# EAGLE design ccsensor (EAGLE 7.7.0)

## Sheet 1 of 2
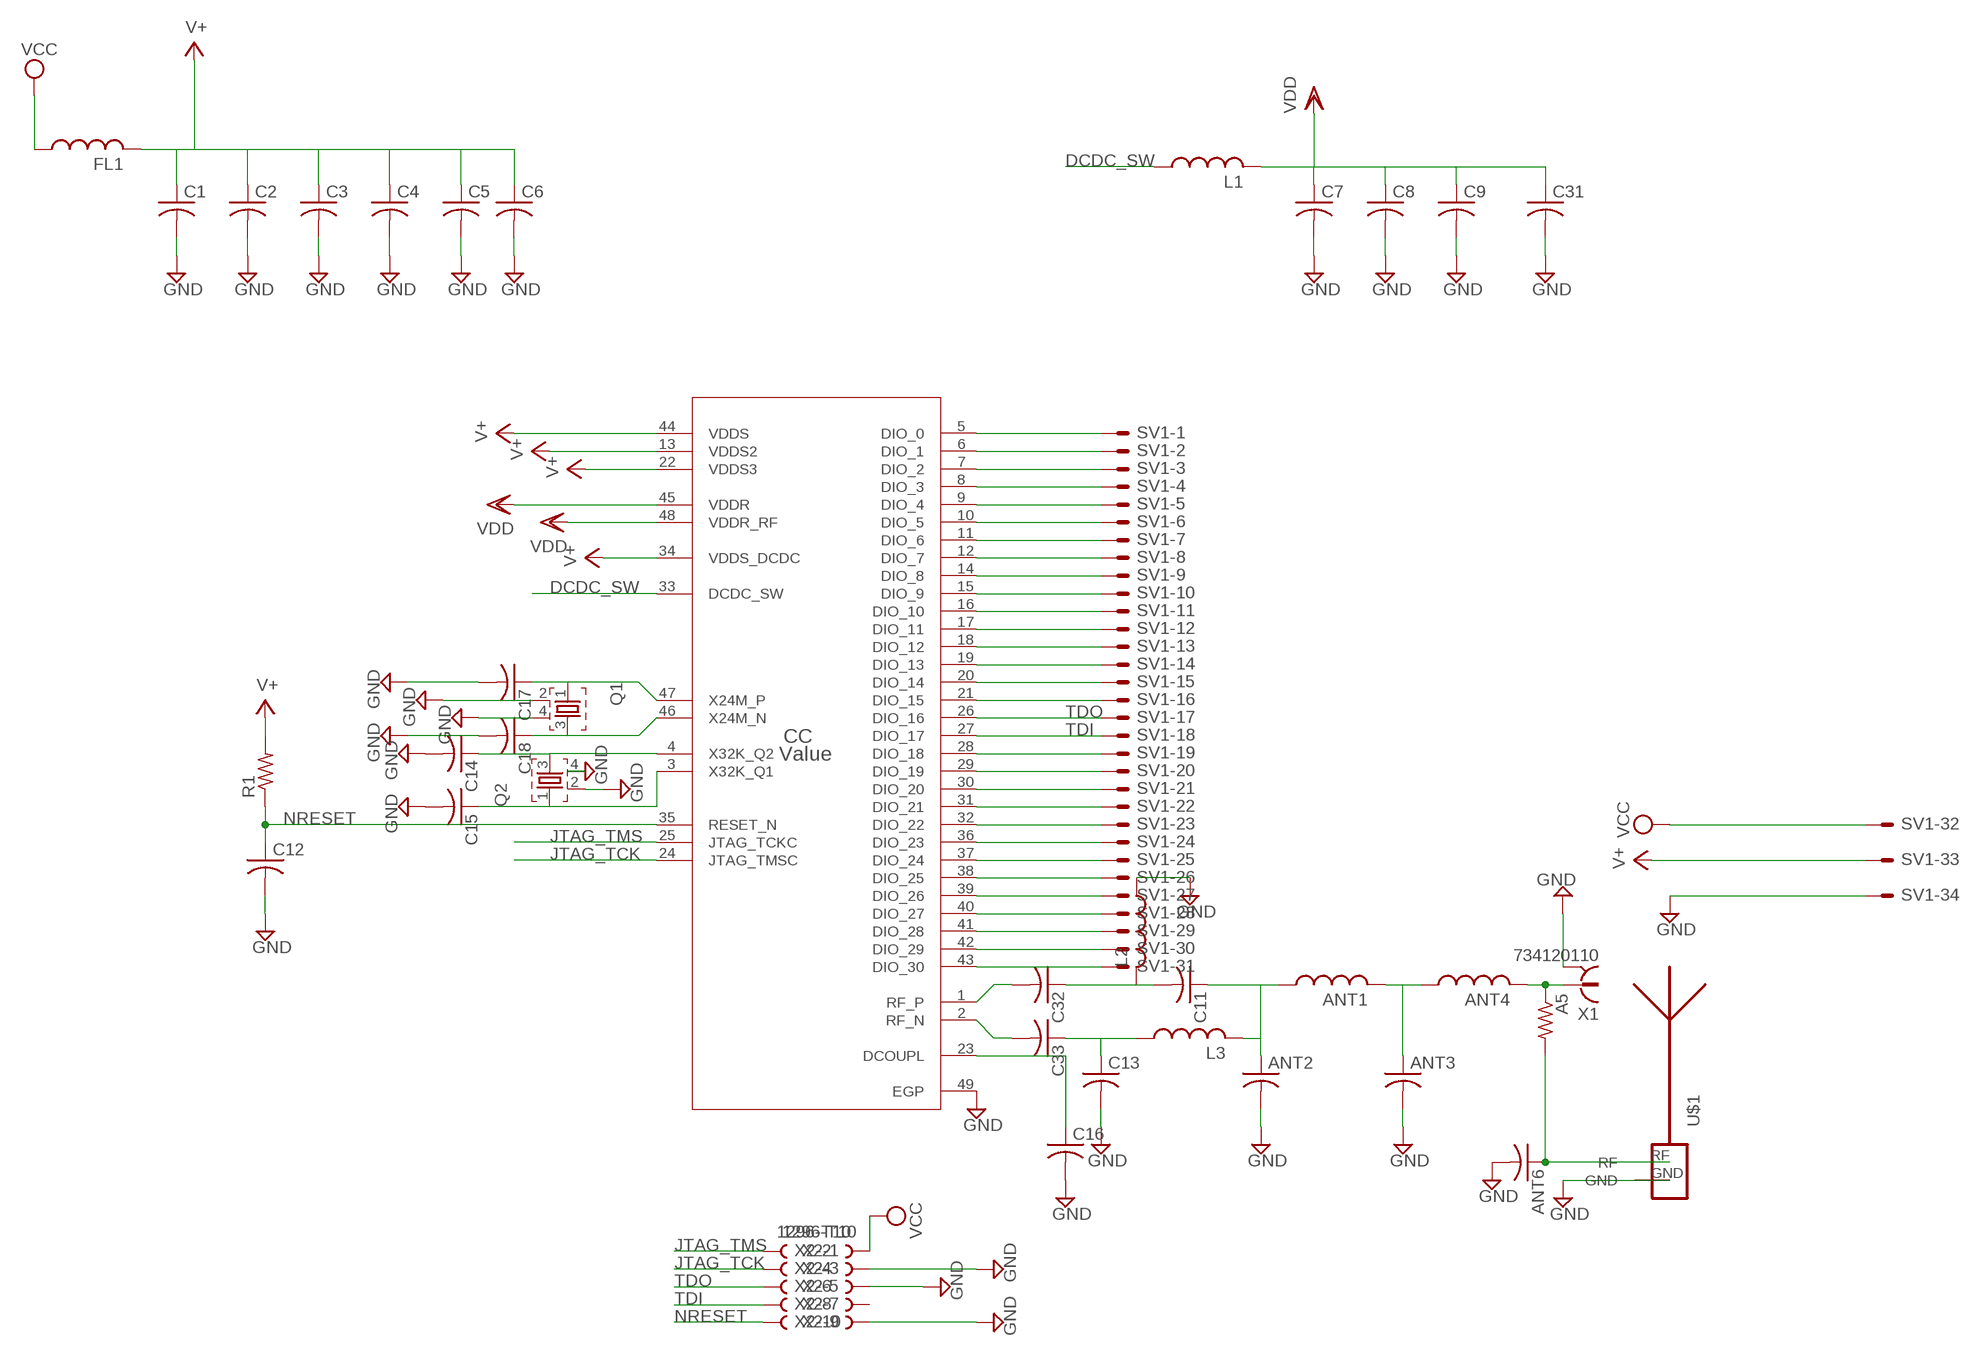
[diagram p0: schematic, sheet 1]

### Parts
A5  R-US_R0402  [R0402]
ANT1  L-USL2012C  [L2012C]
ANT2  C-USC0402  [C0402]
ANT3  C-USC0402  [C0402]
ANT4  L-USL2012C  [L2012C]
ANT6  C-USC0402  [C0402]
C1  C-USC0402  [C0402]
C2  C-USC0402  [C0402]
C3  C-USC0402  [C0402]
C4  C-USC0402  [C0402]
C5  C-USC0603  [C0603]
C6  C-USC0402  [C0402]
C7  C-USC0402  [C0402]
C8  C-USC0402  [C0402]
C9  C-USC0402  [C0402]
C11  C-USC0402  [C0402]
C12  C-USC0402  [C0402]
C13  C-USC0402  [C0402]
C14  C-USC0402  [C0402]
C15  C-USC0402  [C0402]
C16  C-USC0402  [C0402]
C17  C-USC0402  [C0402]
C18  C-USC0402  [C0402]
C31  C-USC0402  [C0402]
C32  C-USC0402  [C0402]
C33  C-USC0402  [C0402]
CC  Value  CC2650F128RGZR  [RGZ0048A]
FL1  L-USL2012C  [L2012C]
L1  L-USL2012C  [L2012C]
L2  L-USL2012C  [L2012C]
L3  L-USL2012C  [L2012C]
Q1  FA-20H  [FA-20H]
Q2  FA-20H  [FA-20H]
R1  R-US_R0402  [R0402]
SV1  ML34E  [ML34]
U$1  ANTENNA_1LEFT  [SWRA117D_LEFT]
X1  734120110  [734120110]
X2  1296-T10  [1296-10]

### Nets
DCDC_SW: CC.33(DCDC_SW) L1.1
GND: ANT2.2 ANT3.2 ANT6.2 C1.2 C2.2 C3.2 C4.2 C5.2 C6.2 C7.2 C8.2 C9.2 C12.2 C13.2 C14.2 C15.2 C16.2 C17.2 C18.2 C31.2 CC.49(EGP) L2.1 Q1.2 Q1.4 Q2.2 Q2.4 SV1.34 U$1.GND X1.S@1 X1.S@2 X1.S@3 X2.3 X2.5 X2.9
JTAG_TCK: CC.24(JTAG_TMSC) X2.4
JTAG_TMS: CC.25(JTAG_TCKC) X2.2
N$1: C18.1 CC.46(X24M_N) Q1.3
N$2: C17.1 CC.47(X24M_P) Q1.1
N$3: C32.2 CC.1(RF_P)
N$4: C15.1 CC.3(X32K_Q1) Q2.1
N$5: C14.1 CC.4(X32K_Q2) Q2.3
N$6: C33.2 CC.2(RF_N)
N$7: C11.2 C32.1 L2.2
N$8: C13.1 C33.1 L3.1
N$9: ANT1.1 ANT2.1 C11.1 L3.2
N$10: ANT1.2 ANT3.1 ANT4.1
N$11: A5.1 ANT4.2 X1.1
N$12: CC.5(DIO_0) SV1.1
N$13: CC.6(DIO_1) SV1.2
N$14: CC.7(DIO_2) SV1.3
N$15: CC.8(DIO_3) SV1.4
N$16: CC.9(DIO_4) SV1.5
N$17: CC.10(DIO_5) SV1.6
N$18: CC.11(DIO_6) SV1.7
N$19: CC.12(DIO_7) SV1.8
N$20: CC.14(DIO_8) SV1.9
N$21: CC.15(DIO_9) SV1.10
N$22: CC.16(DIO_10) SV1.11
N$23: CC.17(DIO_11) SV1.12
N$24: CC.18(DIO_12) SV1.13
N$25: CC.19(DIO_13) SV1.14
N$26: CC.20(DIO_14) SV1.15
N$27: CC.21(DIO_15) SV1.16
N$28: A5.2 ANT6.1 U$1.RF
N$29: C16.1 CC.23(DCOUPL)
N$30: CC.28(DIO_18) SV1.19
N$31: CC.29(DIO_19) SV1.20
N$32: CC.30(DIO_20) SV1.21
N$33: CC.31(DIO_21) SV1.22
N$34: CC.32(DIO_22) SV1.23
N$35: CC.36(DIO_23) SV1.24
N$36: CC.37(DIO_24) SV1.25
N$37: CC.38(DIO_25) SV1.26
N$38: CC.39(DIO_26) SV1.27
N$39: CC.40(DIO_27) SV1.28
N$40: CC.41(DIO_28) SV1.29
N$41: CC.42(DIO_29) SV1.30
N$42: CC.43(DIO_30) SV1.31
NRESET: C12.1 CC.35(RESET_N) R1.1 X2.10
TDI: CC.27(DIO_17) SV1.18 X2.8
TDO: CC.26(DIO_16) SV1.17 X2.6
V+: C1.1 C2.1 C3.1 C4.1 C5.1 C6.1 CC.13(VDDS2) CC.22(VDDS3) CC.34(VDDS_DCDC) CC.44(VDDS) FL1.2 R1.2 SV1.33
VCC: FL1.1 SV1.32 X2.1
VDD: C7.1 C8.1 C9.1 C31.1 CC.45(VDDR) CC.48(VDDR_RF) L1.2
Unconnected: X2.7

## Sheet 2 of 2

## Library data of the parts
A5 R1 = rcl:R-US_: RESISTOR, American symbol; OC_NEWARK: unknown
ANT1 ANT4 FL1 L1-L3 = rcl:L-US: INDUCTOR, American symbol; OC_NEWARK: unknown
ANT2 ANT3 ANT6 C1-C9 C11-C18 C31-C33 = rcl:C-US: CAPACITOR, American symbol; OC_NEWARK: unknown
CC = CC2650F128RGZR:CC2650F128RGZR; ALTERNATEPARTNUMBER: CC2650F128RGZT; APPLICATION_BUILDNUMBER: *; COMPTYPE: IC; MANUFACTURER: Texas Instruments; MOUNTTYPE: SMT; OC_NEWARK: unknown; PACKAGEREFERENCE: RGZ0048A; PARTNUMBER: CC2650F128RGZR; PIN_COUNT: 49; REFDES: RefDes; ROHS: Y; TYPE: TYPE
Q1 Q2 = crystal:FA-: MHz RANGE CRYSTAL UNIT Source: Epson Toyocom; OC_NEWARK: unknown
SV1 = con-ml:ML34E: HARTING; OC_FARNELL: unknown; OC_NEWARK: unknown
U$1 = ant-planar-1:ANTENNA_1; OC_NEWARK: unknown
X1 = con-coax:734120110: MICRO COAXIAL CONNECTOR RECEPTACLE VERTICAL; OC_NEWARK: unknown
X2 = con-leotronics:1296-T10: 1.27mm SINGLE ROW FEMALE SOCKET Source: http://www.leotronics.co.uk/Conexcon/Data%20Sheets/sec.%20A/1296ing.pdf; OC_FARNELL: unknown; OC_NEWARK: unknown

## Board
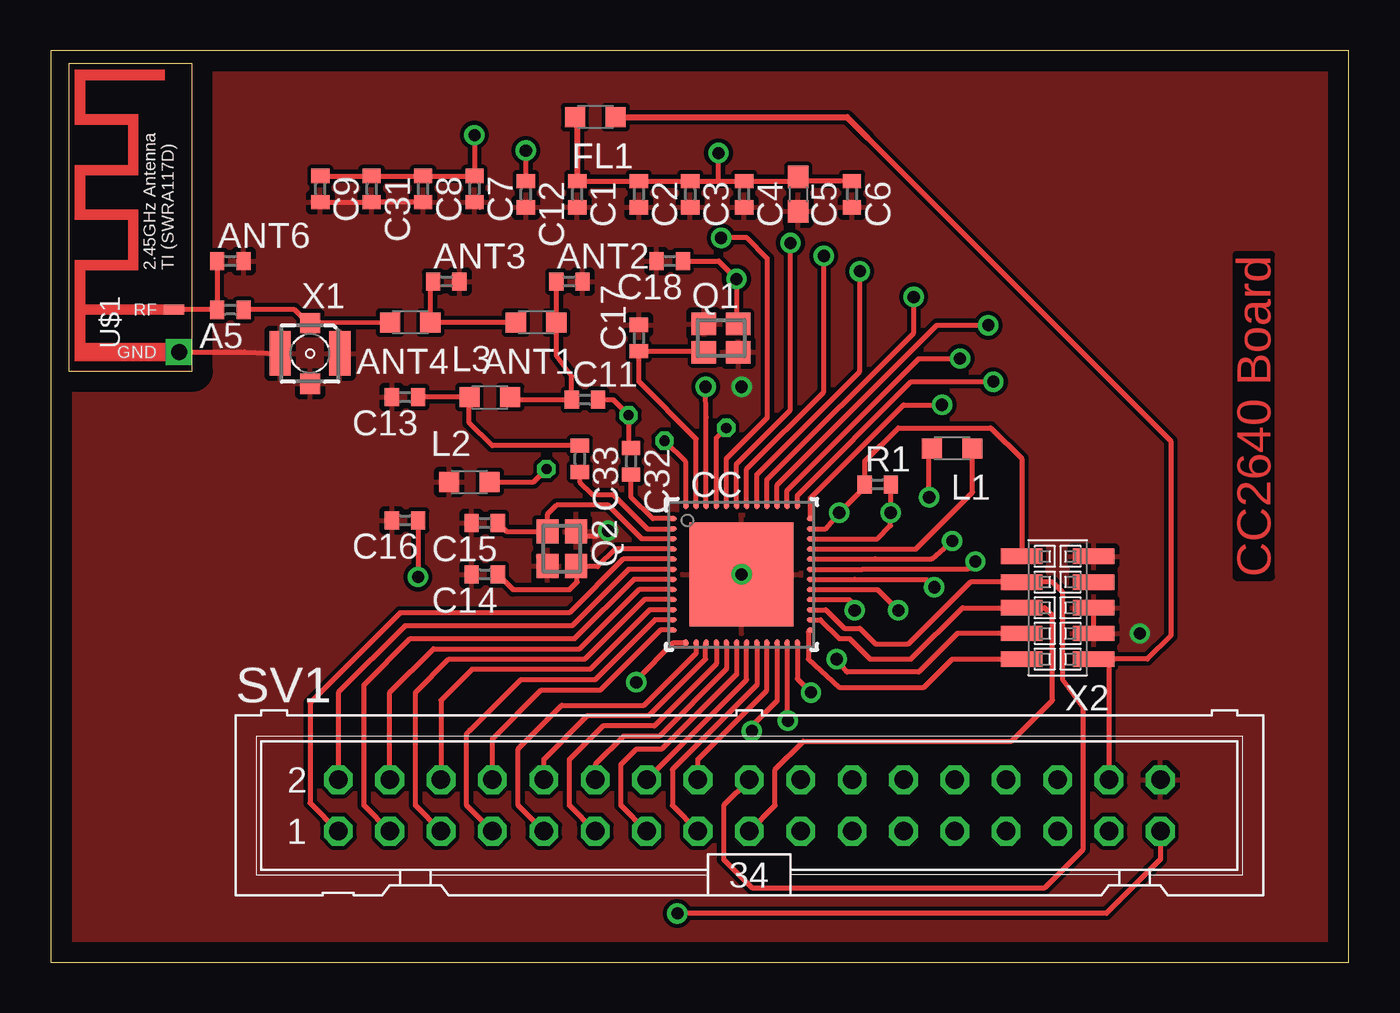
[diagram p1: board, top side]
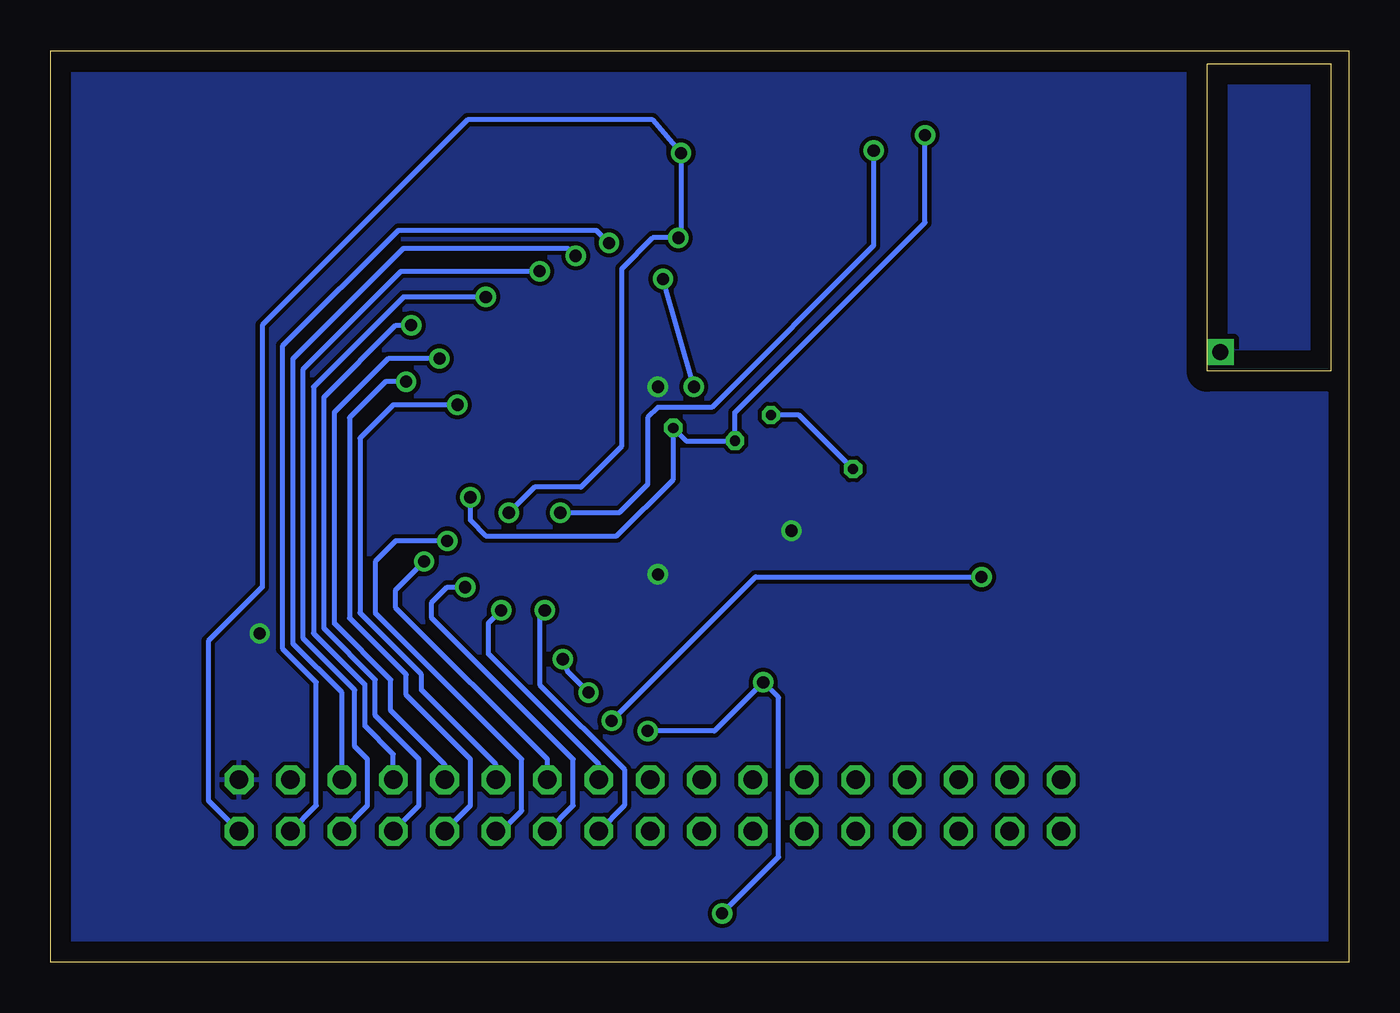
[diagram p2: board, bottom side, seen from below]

Size 64.19 x 45.07 mm. Coordinates in mm from the lower left corner, seen from the top.
Outline: 0,0 64.19,0 64.19,45.07 0,45.07 0,0
Copper layers (1*16): Top 0.035mm / dielectric 1.5mm / Bottom 0.035mm
Design rules "default *": minimum track width 10mil, minimum drill 24mil, track to track 8mil, track to pad 8mil, pad to pad 8mil, via to via 8mil, smd to smd 8mil, copper to edge 40mil, drill to drill 8mil, minimum pad ring 10mil, minimum via ring 8mil, stop-mask expansion 4mil, vias tented up to drill 0mil, thermal gap 10mil

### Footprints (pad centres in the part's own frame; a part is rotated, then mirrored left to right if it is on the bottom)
R0402 = smd 0.7 x 0.9: 1 -0.65,0; 2 0.65,0
L2012C = smd 1 x 1: 1 -1,0; 2 1,0
C0402 = smd 0.7 x 0.9: 1 -0.65,0; 2 0.65,0
C0603 = smd 1.1 x 1: 1 -0.85,0; 2 0.85,0
RGZ0048A = smd 0.36 x 0.24: 1 -3.4,2.75; 2 -3.4,2.25; 3 -3.4,1.75; 4 -3.4,1.25; 5 -3.4,0.75; 6 -3.4,0.25; 7 -3.4,-0.25; 8 -3.4,-0.75; 9 -3.4,-1.25; 10 -3.4,-1.75; 11 -3.4,-2.25; 12 -3.4,-2.75; 25 3.4,-2.75; 26 3.4,-2.25; 27 3.4,-1.75; 28 3.4,-1.25; 29 3.4,-0.75; 30 3.4,-0.25; 31 3.4,0.25; 32 3.4,0.75; 33 3.4,1.25; 34 3.4,1.75; 35 3.4,2.25; 36 3.4,2.75 | smd 0.24 x 0.36: 13 -2.75,-3.4; 14 -2.25,-3.4; 15 -1.75,-3.4; 16 -1.25,-3.4; 17 -0.75,-3.4; 18 -0.25,-3.4; 19 0.25,-3.4; 20 0.75,-3.4; 21 1.25,-3.4; 22 1.75,-3.4; 23 2.25,-3.4; 24 2.75,-3.4; 37 2.75,3.4; 38 2.25,3.4; 39 1.75,3.4; 40 1.25,3.4; 41 0.75,3.4; 42 0.25,3.4; 43 -0.25,3.4; 44 -0.75,3.4; 45 -1.25,3.4; 46 -1.75,3.4; 47 -2.25,3.4; 48 -2.75,3.4 | smd 5.15 x 5.15: 49 0,0 | smd 0.5 x 0.5: V1 -0.803,2.325; V2 0.803,2.325; V3 -2.325,0.803; V4 -0.803,0.803; V5 0.803,0.803; V6 2.325,0.803; V7 -2.325,-0.803; V8 -0.803,-0.803; V9 0.803,-0.803; V10 2.325,-0.803; V11 -0.803,-2.325; V12 0.803,-2.325
FA-20H = smd 1.2 x 1.1: 1 -0.85,-0.7; 2 0.85,-0.7; 3 0.85,0.7; 4 -0.85,0.7
ML34 = drill 0.914 octagon: 1 -20.32,-1.27; 2 -20.32,1.27; 3 -17.78,-1.27; 4 -17.78,1.27; 5 -15.24,-1.27; 6 -15.24,1.27; 7 -12.7,-1.27; 8 -12.7,1.27; 9 -10.16,-1.27; 10 -10.16,1.27; 11 -7.62,-1.27; 12 -7.62,1.27; 13 -5.08,-1.27; 14 -5.08,1.27; 15 -2.54,-1.27; 16 -2.54,1.27; 17 0,-1.27; 18 0,1.27; 19 2.54,-1.27; 20 2.54,1.27; 21 5.08,-1.27; 22 5.08,1.27; 23 7.62,-1.27; 24 7.62,1.27; 25 10.16,-1.27; 26 10.16,1.27; 27 12.7,-1.27; 28 12.7,1.27; 29 15.24,-1.27; 30 15.24,1.27; 31 17.78,-1.27; 32 17.78,1.27; 33 20.32,-1.27; 34 20.32,1.27
SWRA117D_LEFT = drill 0.8 square: GND 0.45,0.25 | smd 0.508 x 1.016: RF 2.55,0.51
734120110 = smd 1 x 1: 1 0,-1.5; S@1 0,1.5 | smd 1.05 x 2.2: S@2 -1.475,0; S@3 1.475,0
1296-10 = smd 0.76 x 2.05: 1 -2.54,-1.78; 2 -2.54,1.78; 3 -1.27,-1.78; 4 -1.27,1.78; 5 0,-1.78; 6 0,1.78; 7 1.27,-1.78; 8 1.27,1.78; 9 2.54,-1.78; 10 2.54,1.78

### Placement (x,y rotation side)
A5  8.89,32.26 180 top
ANT1  24,31.62 180 top
ANT2  25.65,33.66 0 top
ANT3  19.56,33.66 0 top
ANT4  17.78,31.62 180 top
ANT6  8.89,34.67 0 top
C1  26.04,37.97 270 top
C2  29.08,37.97 270 top
C3  31.62,37.97 270 top
C4  34.29,37.97 270 top
C5  36.96,37.97 270 top
C6  39.62,37.97 270 top
C7  20.96,38.23 270 top
C8  18.42,38.23 270 top
C9  13.33,38.23 270 top
C11  26.42,27.81 0 top
C12  23.5,37.97 270 top
C13  17.53,27.94 180 top
C14  21.46,19.18 180 top
C15  21.46,21.72 180 top
C16  17.53,21.84 180 top
C17  29.08,30.86 90 top
C18  30.61,34.67 180 top
C31  15.88,38.23 270 top
C32  28.7,24.77 270 top
C33  26.16,24.89 270 top
CC  34.16,19.18 0 top
FL1  26.92,41.78 180 top
L1  44.58,25.4 180 top
L2  20.7,23.75 0 top
L3  21.72,27.94 0 top
Q1  33.15,30.86 0 top
Q2  25.27,20.45 270 top
R1  40.89,23.62 0 top
SV1  34.54,7.75 0 top
U$1  6.6,29.72 90 top
X1  12.83,30.1 180 top
X2  49.78,17.53 90 top

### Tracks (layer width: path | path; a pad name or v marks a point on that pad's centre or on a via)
DCDC_SW
  Top 0.254: CC.33 42.78,20.43 45.58,23.23 L1.1
GND  (via drill 0.6)
  Top 0.254: Q2.2 24.1,20.07 | C9.2 C31.2 C8.2 | 21.21,37.32 C7.2 | X2.3 X2.5 | 39.64,37.34 C6.2 | U$1.GND 9.57,30.17 X1.S@3 | Q2.4 26.19,21.08 27.05,21.08 v27.56,21.34 | 34.25,28.54 v34.16,28.45
  Bottom 0.254: 34.16,19.05 CC.49 34.16,19.3
  other vias: 53.85,16.26 34.16,19.18
  pour Bottom: 1.02,44.07 0.89,0.38 63.75,0.51 63.75,44.32
  pour Top: 0.64,44.45 0.89,0.38 63.88,0.51 63.88,44.32
JTAG_TCK  (via drill 0.6)
  Top 0.254: v38.86,14.99 39.37,14.35 42.93,14.35 44.83,16.26 X2.4 | CC.24 36.91,14.01 v37.59,13.33
  Bottom 0.254: v37.59,13.33 38.61,14.35 v38.86,14.99
JTAG_TMS
  Top 0.254: CC.25 37.47,16.33 37.47,14.99 38.99,13.59 43.18,13.59 44.58,14.99 X2.2
N$1  (via drill 0.6)
  Top 0.254: Q1.3 33.91,31.65 v33.91,33.78 33.02,34.67 C18.1 | CC.46 32.41,26.95 v32.39,28.45
  Bottom 0.254: v32.39,28.45 v33.91,33.78
N$2
  Top 0.254: 31.91,29.78 Q1.1 32.25,30.21 C17.1 29.08,28.7 31.91,25.87 CC.47
N$3
  Top 0.254: CC.1 29.76,21.93 28.7,22.99 C32.2
N$4
  Top 0.254: C15.1 22.53,21.3 Q2.1 24.57,22.16 25.02,22.61 27.56,22.61 29.24,20.93 CC.3
N$5
  Top 0.254: C14.1 22.87,18.42 | 22.87,18.42 22.88,18.41 | 22.87,18.42 25.66,18.42 26.04,18.8 26.04,19.53 Q2.3 26.01,19.56 27.05,19.56 27.92,20.43 CC.4
N$6
  Top 0.254: 26.29,24.12 C33.2 26.16,23.75 26.8,23.11 27.81,23.11 29.5,21.43 CC.2
N$7  (via drill 0.5)
  Top 0.254: L2.2 23.88,23.75 v24.51,24.38 | C32.1 arc-90 28.57,25.54 v28.57,27.05 27.81,27.81 C11.2
  Bottom 0.254: v24.51,24.38 27.18,27.05 v28.57,27.05
N$8
  Top 0.254: C13.1 L3.1 20.7,27.92 20.7,26.67 21.83,25.54 C33.1
N$9
  Top 0.254: L3.2 22.84,27.81 C11.1 25.77,28.97 25.02,29.97 25.02,31.61 ANT1.1 ANT2.1
N$10
  Top 0.254: ANT3.1 18.78,33.78 ANT4.1 ANT1.2
N$11
  Top 0.254: ANT4.2 X1.1 12.72,31.6 12.07,32.26 A5.1
N$12
  Top 0.254: CC.5 28.31,19.93 25.65,17.27 17.27,17.27 12.83,12.83 12.83,7.87 SV1.1
N$13
  Top 0.254: CC.6 28.57,19.43 25.78,16.64 17.53,16.64 14.22,13.33 SV1.2
N$14
  Top 0.254: CC.7 28.83,18.93 25.91,16 17.78,16 15.49,13.72 15.49,7.75 SV1.3
N$15
  Top 0.254: CC.8 29.1,18.43 26.16,15.49 18.92,15.49 16.76,13.33 SV1.4
N$16
  Top 0.254: CC.9 29.36,17.93 26.42,14.99 19.68,14.99 18.03,13.33 18.03,7.75 SV1.5
N$17
  Top 0.254: CC.10 29.62,17.43 26.67,14.48 20.83,14.48 19.3,12.95 SV1.6
N$18
  Top 0.254: CC.11 29.88,16.93 26.92,13.97 23.24,13.97 20.83,11.56 | SV1.7 20.57,7.75 20.57,11.3 20.83,11.56 | 20.83,11.56 20.7,11.43
N$19
  Top 0.254: CC.12 30.14,16.43 27.18,13.46 24.26,13.46 21.84,11.05 SV1.8
N$20
  Top 0.254: CC.14 31.91,15.28 29.34,12.7 25.27,12.7 23.11,10.54 23.11,7.75 SV1.9
N$21
  Top 0.254: CC.15 32.39,15.75 32.39,14.99 29.59,12.19 26.54,12.19 24.38,10.03 SV1.10
N$22
  Top 0.254: CC.16 32.91,14.75 29.85,11.68 27.31,11.68 25.65,10.03 25.65,7.75 SV1.11
N$23
  Top 0.254: SV1.12 26.92,9.78 28.32,11.18 30.1,11.18 33.41,14.49 CC.17
N$24
  Top 0.254: CC.18 33.91,14.23 30.23,10.54 28.96,10.54 28.19,9.78 28.19,7.75 SV1.13
N$25
  Top 0.254: SV1.14 34.41,13.97 CC.19
N$26
  Top 0.254: CC.20 34.91,13.7 30.73,9.52 30.73,7.75 SV1.15
N$27
  Top 0.254: CC.21 35.41,13.44 32,10.03 SV1.16
N$28
  Top 0.254: U$1.RF A5.2 ANT6.1
N$29  (via drill 0.6)
  Top 0.254: C16.1 18.16,21.73 v18.16,19.05 | CC.23 36.41,11.97 v36.45,11.94
  Bottom 0.254: v36.45,11.94 29.34,19.05 v18.16,19.05
N$30  (via drill 0.6)
  Top 0.254: CC.28 39.48,17.93 39.62,17.78 v39.75,17.4
  Bottom 0.254: v39.75,17.4 40,17.02 40,13.72 35.81,9.52 35.81,7.75 SV1.19
N$31  (via drill 0.6)
  Top 0.254: CC.29 40.88,18.43 v41.91,17.4
  Bottom 0.254: SV1.20 37.08,9.78 42.55,15.24 42.55,16.76 v41.91,17.4
N$32  (via drill 0.6)
  Top 0.254: CC.30 39.75,18.93 41.78,18.92 43.31,18.92 v43.69,18.54
  Bottom 0.254: SV1.21 38.35,7.75 38.35,10.03 45.34,17.02 45.34,17.78 44.58,18.54 v43.69,18.54
N$33  (via drill 0.6)
  Top 0.254: CC.31 40.14,19.43 41.02,19.43 45.34,19.43 v45.72,19.81
  Bottom 0.254: SV1.22 39.62,10.03 47.12,17.53 47.12,18.41 v45.72,19.81
N$34  (via drill 0.6)
  Top 0.254: CC.32 40.27,19.93 40.77,19.94 43.56,19.94 v44.58,20.83
  Bottom 0.254: SV1.23 41.91,6.48 40.89,7.49 40.89,10.03 48.13,17.27 48.13,19.81 47.12,20.83 v44.58,20.83
N$35  (via drill 0.6)
  Top 0.254: v44.07,27.56 42.16,27.56 37.56,22.96 CC.36
  Bottom 0.254: SV1.24 42.16,9.78 45.85,13.46 45.85,14.22 48.89,17.27 48.89,25.91 47.24,27.56 v44.07,27.56
N$36  (via drill 0.6)
  Top 0.254: CC.37 36.91,23.07 42.55,28.7 v46.61,28.7
  Bottom 0.254: SV1.25 43.43,7.75 43.43,10.03 46.61,13.21 46.61,14.22 49.4,17.02 49.4,26.92 47.62,28.7 v46.61,28.7
N$37  (via drill 0.6)
  Top 0.254: CC.38 36.41,23.33 42.93,29.84 v44.96,29.84
  Bottom 0.254: SV1.26 44.7,9.78 47.37,12.45 47.37,13.97 50.16,16.76 50.16,27.18 47.5,29.84 v44.96,29.84
N$38  (via drill 0.6)
  Top 0.254: v46.36,31.5 43.81,31.5 35.91,23.59 CC.39
  Bottom 0.254: SV1.27 45.97,7.75 45.97,10.03 48.13,12.19 48.13,13.97 50.67,16.51 50.67,27.94 47.12,31.5 v46.36,31.5
N$39  (via drill 0.6)
  Top 0.254: CC.40 35.41,23.86 42.67,31.12 v42.67,32.89
  Bottom 0.254: v42.67,32.89 46.74,32.89 51.18,28.45 51.18,16.26 48.64,13.72 48.64,11.68 47.24,10.29 SV1.28
N$40  (via drill 0.6)
  Top 0.254: CC.41 34.91,24.12 40,29.21 v40,34.16
  Bottom 0.254: SV1.29 48.51,7.75 48.51,10.03 49.15,10.67 49.15,13.46 51.69,16 51.69,29.34 46.86,34.16 v40,34.16
N$41  (via drill 0.6)
  Top 0.254: CC.42 34.41,24.38 38.23,28.19 v38.23,34.92
  Bottom 0.254: v38.23,34.92 38.61,35.31 46.74,35.31 52.2,29.84 52.2,15.75 49.78,13.33 SV1.30
N$42  (via drill 0.6)
  Top 0.254: CC.43 33.91,24.64 36.58,27.3 v36.58,35.56
  Bottom 0.254: SV1.31 51.05,7.75 51.05,13.84 52.7,15.49 52.7,30.48 46.99,36.2 37.21,36.2 v36.58,35.56
NRESET  (via drill 0.6)
  Top 0.254: CC.35 38.32,21.43 v38.99,22.23 | C12.1 v23.5,40.13 | v38.99,22.23 v38.99,22.24 | X2.10 48.01,24.89 46.48,26.42 41.91,26.42 40.24,24.75 R1.1 40.24,23.48 v38.99,22.23
  Bottom 0.254: v23.5,40.13 23.5,35.43 31.5,27.43 34.16,27.43 34.67,26.92 34.67,23.62 36.07,22.23 v38.99,22.23
TDI
  Top 0.254: SV1.18 33.27,7.75 33.27,5.08 34.67,3.68 49.15,3.68 51.05,5.59 51.05,12.57 50.04,13.97 50.04,18.29 49.53,18.8 X2.8 45.47,18.8 42.42,15.75 40.77,15.75 40,16.51 39.24,16.51 38.33,17.43 CC.27
TDO
  Top 0.254: SV1.17 35.81,7.75 35.81,9.52 37.21,10.92 47.5,10.92 49.53,12.95 49.53,17.14 49.15,17.53 X2.6 45.08,17.53 42.55,14.99 40.51,14.99 39.5,16 38.99,16 38.06,16.93 CC.26
V+  (via drill 0.6)
  Top 0.254: C1.1 C2.1 C3.1 33.02,38.62 | 33.02,38.62 C4.1 36.96,38.62 | 33.02,38.62 v33.02,40 | CC.13 30.76,15.78 28.96,13.97 v28.96,13.84 | SV1.33 54.86,5.08 52.2,2.41 v30.99,2.41 | 41.53,23.61 R1.2 v41.54,22.24 v41.53,22.23 41.53,21.59 40.87,20.93 CC.34 | C6.1 36.96,38.62 | 36.96,38.62 C5.1 | v34.67,11.43 34.67,11.68 35.91,12.93 CC.22 | v33.15,35.81 34.42,35.81 35.43,34.8 35.43,26.92 33.41,24.9 CC.44
  Top 0.305: FL1.2 26.04,41.78 C1.1
  Bottom 0.254: v30.99,2.41 28.19,5.21 28.19,13.08 v28.96,13.84 31.37,11.43 v34.67,11.43 | SV1.33 56.39,8 56.39,15.88 53.72,18.54 53.72,31.5 43.56,41.66 34.42,41.66 v33.02,40 33.02,35.94 v33.15,35.81 34.42,35.81 35.94,34.29 35.94,25.53 37.97,23.49 40.26,23.49 v41.53,22.23
VCC
  Top 0.254: 40.39,40.77 55.37,25.78 55.37,16.13 54.23,14.99 52.58,14.99 52.32,14.73 | X2.1 52.32,14.99 52.32,14.73 | 52.32,14.73 SV1.32
  Top 0.305: FL1.1 39.37,41.78 40.39,40.77
VDD  (via drill 0.5, 0.6)
  Top 0.254: C9.1 C31.1 C8.1 C7.1 v20.96,40.89 | v43.43,22.99 43.43,25.4 L1.2 | CC.48 31.41,24.72 v30.35,25.78 | v33.4,26.42 32.91,25.93 CC.45
  Bottom 0.254: v20.96,40.89 20.96,36.58 30.35,27.18 v30.35,25.78 32.77,25.78 v33.4,26.42 33.4,23.88 36.2,21.08 42.67,21.08 43.43,21.84 v43.43,22.99

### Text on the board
Top: CC2640 Board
